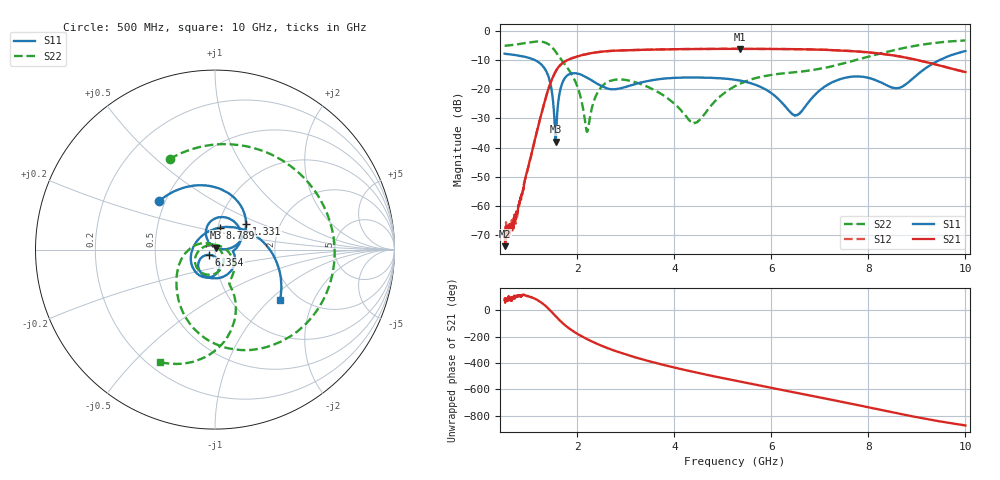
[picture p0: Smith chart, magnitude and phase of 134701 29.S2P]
!  2-Port S-parameters saved by WinCal
! VAR MeasName=S-Parameters (CALIBRATED_DATA) read from VNA (N5242A)
! VAR MeasDate=2013-7-3 16:33:04
! VAR NAME=134701 29
! VAR FILENAME=134701 29.S2P
! VAR DATE=2013-7-3 16:33:04
! VAR PHYS_PORTS=1,2
# Hz S MA R 50
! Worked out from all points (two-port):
!   1601 points, 500 MHz to 10 GHz, reference 50 ohm
!   highest |S21| = -6.02 dB at 5.345 GHz (marker M1); lowest = -74.0 dB at 511.9 MHz (marker M2)
!   |S21| within 3 dB of the highest: 1.929 GHz to 8.762 GHz (6.833 GHz wide, 128 % of centre)
!   lowest |S11| = -37.9 dB at 1.551 GHz (marker M3), VSWR 1.03, Z = 50.5 + j1.15 ohm
!   |S11| at or under -10 dB: 1.139 GHz to 9.452 GHz (8.313 GHz wide, 157 % of centre)
!   |S22| runs from -34.6 to -3.1 dB; largest |S21 - S12| = 0.0024
!   S11 on the Smith chart (normalised r, x): 500 MHz: 0.46, +0.30; 1.331 GHz: 1.35, +0.41; 6.354 GHz: 0.94, -0.05; 8.789 GHz: 1.02, +0.25; 10 GHz: 1.63, -1.16
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5e8  0.4121 139.2  0.0003775 75.8  0.0003079 46.7  0.5645 116.6
5.11875e8  0.4112 138.3  0.0002004 55.1  0.000266 61.2  0.5656 114.9
6.840625e8  0.3944 123.5  0.0004128 100.8  0.0006106 101.5  0.586 89.4
9.15625e8  0.3652 100.9  0.00265 111.4  0.002718 111.9  0.6263 49.3
1.147188e9  0.3135 72.0  0.01606 81.3  0.01611 81.6  0.6662 0.2
1.33125e9  0.2254 39.8  0.06394 35.2  0.06409 35.1  0.6434 -47.0
1.550938e9  0.01267 64.1  0.2032 -45.8  0.2031 -45.8  0.4479 -106.4
1.729062e9  0.1508 102.6  0.298 -109.6  0.2977 -109.6  0.2786 -140.5
2.085312e9  0.179 39.9  0.3883 162.5  0.3882 162.5  0.06363 145.3
2.21e9  0.1579 24.3  0.4095 138.4  0.41 138.5  0.01894 38.3
2.625625e9  0.1035 -3.1  0.4568 71.8  0.4572 71.7  0.1352 -90.7
3.118438e9  0.1187 -20.6  0.4755 10.8  0.4755 10.7  0.1387 -140.4
3.670625e9  0.1499 -55.2  0.4879 -44.8  0.4875 -44.8  0.08941 -176.4
4.41875e9  0.1603 -93.0  0.4966 -109.4  0.4976 -109.4  0.02626 81.0
5.25e9  0.1467 -124.8  0.4994 -173.6  0.5 -173.7  0.114 -28.8
5.345e9  0.1425 -128.4  0.4999 179.4  0.4998 179.2  0.1247 -33.6
6.354375e9  0.04372 -138.3  0.4946 106.3  0.4951 106.3  0.1933 -64.8
6.835312e9  0.0707 -73.0  0.4885 71.6  0.4886 71.6  0.2147 -67.5
7.60125e9  0.1637 -108.1  0.4608 15.3  0.461 15.1  0.2975 -67.9
8.420625e9  0.1136 159.7  0.3954 -46.6  0.3941 -46.8  0.4509 -78.2
8.78875e9  0.1255 77.3  0.3507 -74.1  0.3503 -74.3  0.5294 -85.8
1e10  0.4581 -37.6  0.1993 -151.9  0.1989 -151.8  0.697 -116.0
